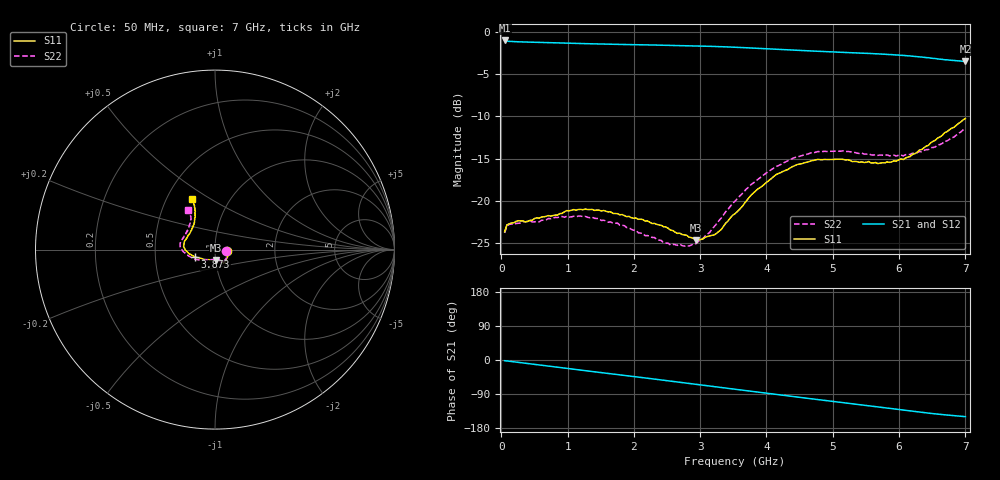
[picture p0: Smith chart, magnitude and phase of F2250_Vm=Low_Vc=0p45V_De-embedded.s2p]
! Integrated Device Technology
! Corporate Headquarters
! 6024 Silver Creek Valley Road
! San Jose, CA 95138  USA
! Phone:  1-408-284-8200
! Toll Free:  1-800-223-1366
! Webpage:  http://www.idt.com/
! Timing and RF Division
! 515 Groton Road, Suite 102
! Westford, MA 01886-6024
! Device:  F2250
! Description: Voltage Variable RF Attenuator
! Frequency:  50.0 -  6000.00 MHz
! Package:  3x3 mm Thin QFN Plastic Package: 16 pin
! Ports:  2 RF, 3 DC
!  Pin  1  = GND
!  Pin  2  = NC
!  Pin  3  = RF1  = Port 1
!  Pin  4  = NC
!  Pin  5  = GND
!  Pin  6  = GND
!  Pin  7  = GND
!  Pin  8  = GND
!  Pin  9  = NC
!  Pin 10  = RF2  = Port 2
!  Pin 11  = NC
!  Pin 12  = GND
!  Pin 13  = GND
!  Pin 14  = VCNTRL
!  Pin 15  = VDD
!  Pin 16  = VMODE
! Vcntrl:  0.450 Volts
! Vmode:  +0.000 Volts
! Vdd:  +3.30  Volts
! Current:  1.127 mA
! Data:  The device was measured on a the F2250 evaluation board which has
!  individual transmission lines to the RF pins.  Data was collected
!  using a calibrated network analyzer.  The evaluation board was
!  de-embedded using a TRL calibration technique.
!  The reference plane is the edge of the package pin.
! Misc:  SN 10
!  Action Tracker AT0258
! Date Measured:  2014-11-26
! Date:  2015-10-15  MJV
! Note:
!  Integrated Device Technology supplies this data as a sample of measured
!  data at the package pin for this product.  Your particular data for this
!  product may vary.
!  Data was taken at 25 degrees C.
!  Integrated Device Technology reserves the right to change this data at anytime.
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# GHz S dB R 50
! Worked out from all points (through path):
!   201 points, 50 MHz to 7 GHz, reference 50 ohm
!   highest |S21| = -1.03 dB at 50 MHz (marker M1); lowest = -3.5 dB at 7 GHz (marker M2)
!   group delay of S21, straight-line fit = 60.1 ps
!   lowest |S11| = -24.6 dB at 2.934 GHz (marker M3), VSWR 1.12, Z = 50.2 - j5.88 ohm
!   |S11| at or under -10 dB: start of sweep to end of sweep
!   |S22| runs from -25.4 to -11.4 dB; largest |S21 - S12| = 0.00037
!   S11 on the Smith chart (normalised r, x): 50 MHz: 1.14, -0.02; 3.873 GHz: 0.80, -0.07; 7 GHz: 0.67, +0.42
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0.05  -23.64 -8.4  -1.03 -1.8  -1.03 -1.8  -23.80 -9.1
0.08475  -22.84 -8.3  -1.10 -2.5  -1.10 -2.5  -22.94 -8.4
0.15425  -22.62 -10.4  -1.15 -4.0  -1.15 -4.0  -22.73 -10.2
0.6755  -21.83 -32.7  -1.28 -15.4  -1.28 -15.4  -22.25 -34.4
0.884  -21.51 -41.6  -1.32 -20.0  -1.32 -20.0  -21.87 -44.4
1.2315  -21.05 -51.5  -1.40 -27.4  -1.40 -27.4  -21.88 -57.1
1.75275  -21.52 -58.2  -1.49 -38.5  -1.49 -38.5  -22.62 -65.2
2.37825  -22.85 -59.5  -1.58 -51.8  -1.58 -51.8  -24.65 -69.8
2.552  -23.46 -63.3  -1.60 -55.6  -1.60 -55.7  -25.23 -75.5
2.93425  -24.65 -84.3  -1.67 -64.0  -1.67 -64.0  -25.07 -101.1
3.21225  -24.03 -112.3  -1.74 -70.2  -1.73 -70.2  -23.03 -125.2
3.525  -21.53 -140.8  -1.83 -77.2  -1.83 -77.2  -20.03 -144.2
3.8725  -18.57 -159.1  -1.96 -84.8  -1.96 -84.8  -17.44 -159.9
4.1505  -16.87 -169.7  -2.07 -90.9  -2.07 -90.9  -15.93 -170.0
4.4285  -15.83 -177.7  -2.18 -96.9  -2.18 -96.9  -14.87 -177.3
4.7065  -15.22 175.4  -2.28 -102.9  -2.28 -103.0  -14.33 176.5
5.15825  -15.10 164.5  -2.44 -112.7  -2.44 -112.7  -14.08 167.1
5.85325  -15.44 141.0  -2.69 -127.6  -2.69 -127.6  -14.68 151.8
6.166  -14.76 129.8  -2.86 -134.4  -2.86 -134.4  -14.51 142.8
6.444  -13.43 121.0  -3.07 -140.2  -3.07 -140.2  -13.93 133.4
6.82625  -11.31 115.0  -3.39 -146.9  -3.39 -146.9  -12.47 125.4
7  -10.26 114.2  -3.51 -149.5  -3.51 -149.5  -11.45 123.9
